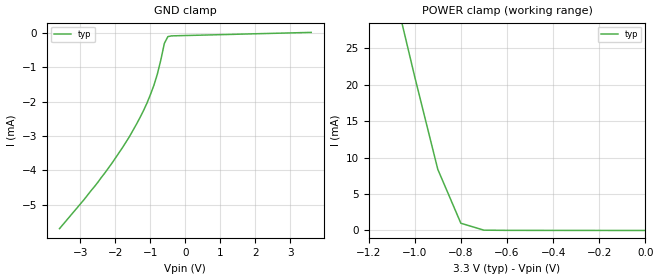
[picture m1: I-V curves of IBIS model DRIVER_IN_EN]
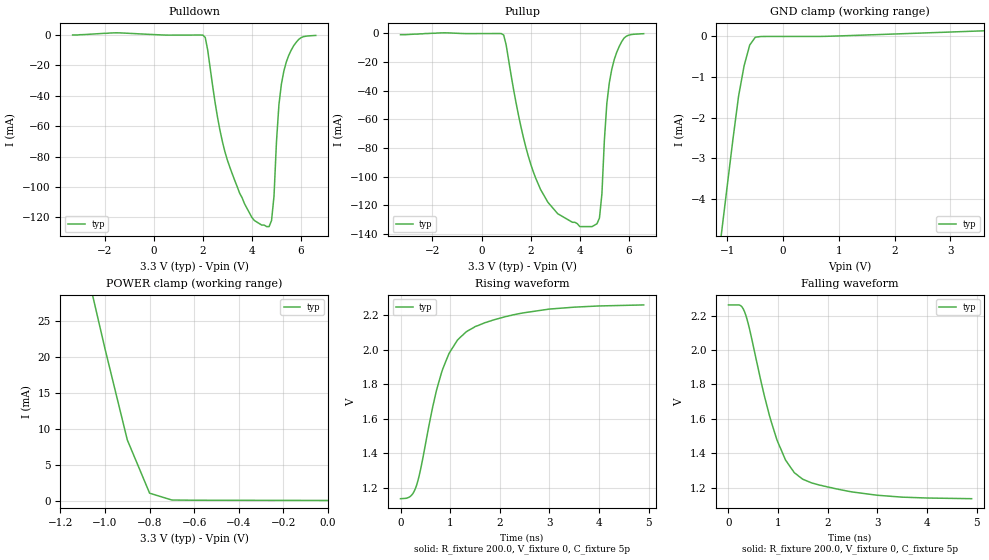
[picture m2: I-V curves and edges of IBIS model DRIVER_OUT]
|   Texas Instruments Incorporated
|   Data Transmissions Products
|   IBIS Model for TB5D1M
|   16D SOIC Package
[IBIS Ver]   3.2
[Comment char]   |_char
[File name]   tb5d1m3vd.ibs
[File Rev]   1.0
[Date]   14Apr03
[Source]   File originated at Texas Instruments Incorporated.
   Data Transmission Products Group. All data based on
   Simulation.
[Notes]  Model for 3V operation.
[Disclaimer]
(C) Copyright Texas Instruments Incorporated 2003
   All rights reserved
  Texas Instruments Incorporated hereby grants the user of this IBIS
model a non-exclusive, nontransferable license to use this IBIS model
under the following terms.  Before using this IBIS model, the user
should read this license.  If the user does not accept these terms,
the IBIS model should be returned to Texas Instruments within 30 days.
  The user is granted this license only to use the IBIS model and
is not granted rights to sell, load, rent, lease or license the IBIS
model in whole or in part, or in modified form to anyone other than
user.  User may modify the IBIS model to suit its specific applications
but rights to derivative works and such modifications shall belong to
Texas Instruments.
  This IBIS model is provided on an "AS IS" basis and Texas Instruments
makes absolutely no warranty with respect to the information contained
herein.  TEXAS INSTRUMENTS DISCLAIMS AND CUSTOMER WAIVES ALL WARRANTIES,
EXPRESS OR IMPLIED, INCLUDING WARRANTIES OF MERCHANTABILITY OR FITNESS
FOR A PARTICULAR PURPOSE. The entire risk as to quality and performance
is with the Customer. ACCORDINGLY, IN NO EVENT SHALL THE COMPANY BE LIABLE
FOR ANY DAMAGES, WHETHER IN CONTRACT OR TORT,INCLUDING ANY LOST PROFITS
OR OTHER INCIDENTAL, CONSEQUENTIAL, EXEMPLARY, OR PUNITIVE DAMAGES ARISING
OUT OF THE USE OR APPLICATION OF THE IBIS model provided in this package.
Further, Texas Instruments reserves the right to discontinue or make changes
without notice to any product herein to improve reliability, function, or
design. Texas Instruments does not convey any license under patent rights
or any other intellectual property rights, including those of third parties.
Contact Texas Instruments at ATTN:DATA TRANSMISSIONS
[Copyright]   Copyright 2003, Texas Instruments, All Rights Reserved
[Component]   TB5D1M
[Manufacturer]  Texas Instruments
[Package]
|   typ   min   max
R_pkg   0.035   0.030   0.040
L_pkg   2.181nH   1.231nH   3.257nH
C_pkg   0.322pF   0.163pF   0.546pF
[Pin]   signal_name   model_name   R_pin   L_pin   C_pin
1   AI   DRIVER_IN_EN   0.040   3.251n   0.546p
2   AO   DRIVER_OUT   0.039   2.561n   0.393p
3   AO(-)   DRIVER_OUT   0.030   1.681n   0.186p
4   E1   DRIVER_IN_EN   0.030   1.231n   0.163p
5   BO(-)   DRIVER_OUT   0.030   1.231n   0.163p
6   BO   DRIVER_OUT   0.030   1.681n   0.186p
7   BI   DRIVER_IN_EN   0.039   2.564n   0.393p
8   GND   GND   0.040   3.257n   0.545p
9   CI   DRIVER_IN_EN   0.040   3.247n   0.546p
10   CO   DRIVER_OUT   0.039   2.558n   0.394p
11   CO(-)   DRIVER_OUT   0.030   1.681n   0.187p
12   E2   DRIVER_IN_EN   0.030   1.231n   0.163p
13   DO(-)   DRIVER_OUT   0.030   1.231n   0.163p
14   DO   DRIVER_OUT   0.030   1.681n   0.187p
15   DI   DRIVER_IN_EN   0.039   2.558n   0.394p
16   VCC   POWER   0.040   3.246n   0.546p
[Diff_pin]   inv_pin   vdiff   tdelay_typ   tdelay_min   tdelay_max
| The 'AO(+) (or 'xO(+)')' and inv_pins, 'AO(-) (or 'xO(-)')', pins
| are Diff_pins
   2   3   0   0   0   0
   6   5   0   0   0   0
   10   11   0   0   0   0
   14   13   0   0   0   0
| Models and submodels in the file (2): DRIVER_IN_EN (Input), DRIVER_OUT (Output_ECL)
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|   Driver Input Model
[Model]   DRIVER_IN_EN
Model_type   Input
|Signals   AI,BI,CI,DI,E1,E2
Vinh = 2.4
Vinl = 0.4
|   typ   min   max
C_comp   1.03pF   NA   NA
|   typ   min   max
[Temperature Range]   25.0   NA   NA
[Voltage range]   3.3V   NA   NA
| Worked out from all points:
|   GND clamp passes 1 mA (typ) near -0.75 V on its own axis
|   POWER clamp passes 1 mA (typ) near -0.80 V on its own axis
[GND_clamp]
| Voltage   I(typ)   I(min)   I(max)
-3.6V     -5.69mA    NA         NA
-2.5V     -4.34mA    NA         NA
-2.1V     -3.79mA    NA         NA
-1.6V     -3.02mA    NA         NA
-1.2V     -2.27mA    NA         NA
-1V       -1.8mA     NA         NA
-900mV    -1.53mA    NA         NA
-800mV    -1.2mA     NA         NA
-700mV    -787uA     NA         NA
-600mV    -309uA     NA         NA
-500mV    -114uA     NA         NA
3.6V      8.57uA     NA         NA
[Power_clamp]
| Note that the[POWER_clamp]voltage table is referenced to Vcc
| and is calculated using Vtable=Vcc - Vmeasured.
|   Voltage   I(typ)   I(min)   I(max)
-3.3V     147mA      NA         NA
-1.1V     34.4mA     NA         NA
-1V       21.1mA     NA         NA
-900mV    8.39mA     NA         NA
-800mV    993uA      NA         NA
-700mV    43.8uA     NA         NA
0V        1.05uA     NA         NA
|   Driver Output Model
[Model]   DRIVER_OUT
|Model_type   3-state_ECL
Model_type   Output_ECL
| Signals   O(+),O(-)
Vmeas = 1.8V   |Reference voltage for timing measurements
Cref = 5pF   |Timing specification test load capacitance value
Rref = 200   |Note: 200 Ohm load; single ended configuration
| variable   typ   min   max
C_comp   958fF   NA   NA
|   typ   min   max
[Temperature Range]   25.0   NA   NA
[Voltage range]   3.3V   NA   NA
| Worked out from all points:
|   GND clamp passes 1 mA (typ) near -0.74 V on its own axis
|   POWER clamp passes 1 mA (typ) near -0.79 V on its own axis
|   rising waveform, R_fixture 200.0, V_fixture 0, C_fixture 5p: 20-80 % time 658ps typ, NA min, NA max; typ from 1.14 V to 2.26 V
|   falling waveform, R_fixture 200.0, V_fixture 0, C_fixture 5p: 20-80 % time 659ps typ, NA min, NA max; typ from 2.26 V to 1.14 V
[Pulldown]
|   Voltage   I(typ)   I(min)   I(max)
-3.3V     0A         NA         NA
2.1V      -1.6mA     NA         NA
2.6V      -54.1mA    NA         NA
3V        -82.2mA    NA         NA
4V        -120mA     NA         NA
4.6V      -126mA     NA         NA
4.8V      -122mA     NA         NA
4.9V      -106mA     NA         NA
5.1V      -45.9mA    NA         NA
5.3V      -23.8mA    NA         NA
5.9V      -3mA       NA         NA
6.6V      -300uA     NA         NA
[Pullup]
|   Voltage   I(typ)   I(min)   I(max)
| Note that the[Pullup]voltage table is referenced to Vcc
| and is calculated using Vtable=Vcc - Vmeasured.
-3.3V     -900uA     NA         NA
900mV     -1.15mA    NA         NA
1.7V      -72.5mA    NA         NA
2.4V      -109mA     NA         NA
3.1V      -126mA     NA         NA
4.5V      -135mA     NA         NA
4.8V      -129mA     NA         NA
4.9V      -112mA     NA         NA
5.1V      -49mA      NA         NA
5.4V      -18.4mA    NA         NA
5.8V      -3.3mA     NA         NA
6.6V      -200uA     NA         NA
[GND_clamp]
|   Voltage   I(typ)   I(min)   I(max)
| Outputs in High Impedance (off)
-3.6V     -165mA     NA         NA
-1.1V     -4.77mA    NA         NA
-900mV    -2.52mA    NA         NA
-800mV    -1.47mA    NA         NA
-700mV    -718uA     NA         NA
-600mV    -212uA     NA         NA
-500mV    -19.1uA    NA         NA
-400mV    -976nA     NA         NA
800mV     4.54uA     NA         NA
3.6V      139uA      NA         NA
[Power_clamp]
| Note that the[POWER_clamp]voltage table is referenced to Vcc
| and is calculated using Vtable=Vcc - Vmeasured.
|   Voltage   I(typ)   I(min)   I(max)
-3.3V     150mA      NA         NA
-1.1V     34.4mA     NA         NA
-1V       21.1mA     NA         NA
-900mV    8.5mA      NA         NA
-800mV    1.13mA     NA         NA
-700mV    183uA      NA         NA
0V        124uA      NA         NA
[Ramp]
|   typ   min   max
dV/dt_r   0.676/662pS   NA   NA
dV/dt_f   0.676/659pS   NA   NA
R_load = 200ohm
[Rising Waveform]
R_fixture = 200.0
V_fixture = 0
C_fixture = 5p
|   V(typ)   V(min)   V(max)
0s        1.138V     NA         NA
175ps     1.147V     NA         NA
300ps     1.197V     NA         NA
400ps     1.302V     NA         NA
650ps     1.672V     NA         NA
825ps     1.867V     NA         NA
1.025ns   2.002V     NA         NA
1.325ns   2.105V     NA         NA
2.5ns     2.216V     NA         NA
4.9ns     2.261V     NA         NA
[Falling Waveform]
R_fixture = 200.0
V_fixture = 0
C_fixture = 5p
|   V(typ)   V(min)   V(max)
0s        2.262V     NA         NA
225ps     2.261V     NA         NA
325ps     2.222V     NA         NA
725ps     1.732V     NA         NA
975ps     1.479V     NA         NA
1.15ns    1.36V      NA         NA
1.35ns    1.281V     NA         NA
1.675ns   1.227V     NA         NA
2.5ns     1.174V     NA         NA
4.9ns     1.135V     NA         NA
